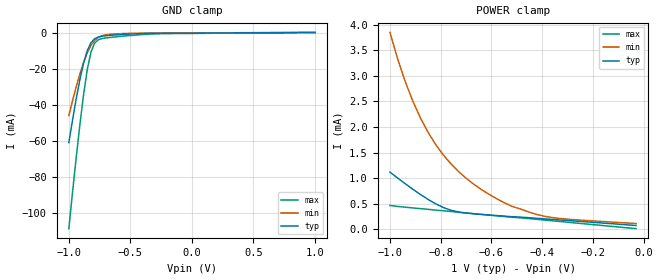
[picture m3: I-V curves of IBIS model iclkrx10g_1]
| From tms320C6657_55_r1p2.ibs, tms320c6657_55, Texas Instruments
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|   Model Cell iclkrx10g_1
|iclkrx10g_1  [08July11 revision 1.3]
[Model]   iclkrx10g_1
Model_type   Input
Polarity   Non-Inverting
Vinl =  1.15
Vinh =  1.25
C_comp   5.02654p   4.29394p   6.16252p
[Model Spec]
Vinl   1.15   1.15   1.15
Vinh   1.25   1.25   1.25
[Temperature Range]   25   125   -40
[Voltage Range]   1   0.9   1.1
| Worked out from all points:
|   GND clamp passes 1 mA (typ) near -0.56 V on its own axis
|   POWER clamp passes 1 mA (typ) near -0.97 V on its own axis
[GND_clamp]
|   voltage   I(typ)   I(min)   I(max)
-1V       -60.88mA   -45.91mA   -108.5mA
-940mV    -36.6mA    -29.97mA   -69.05mA
-910mV    -25.93mA   -22.84mA   -50.79mA
-880mV    -16.82mA   -16.48mA   -34.22mA
-850mV    -9.913mA   -11.15mA   -20.37mA
-820mV    -5.577mA   -7.06mA    -10.7mA
-790mV    -3.405mA   -4.281mA   -5.775mA
-760mV    -2.454mA   -2.625mA   -3.962mA
-700mV    -1.754mA   -1.25mA    -2.986mA
-640mV    -1.394mA   -811.8uA   -2.514mA
-300mV    -411.2uA   -270.4uA   -717.9uA
1V        64.27uA    104.3uA    -1.417uA
[POWER_clamp]
|   voltage   I(typ)   I(min)   I(max)
-1V       1.118mA    3.85mA     465.3uA
-970mV    1.004mA    3.34mA     447.5uA
-940mV    892.4uA    2.894mA    432.6uA
-910mV    784.7uA    2.509mA    418.3uA
-850mV    585.7uA    1.899mA    390.2uA
-820mV    499.2uA    1.66mA     376.2uA
-760mV    373uA      1.282mA    348.1uA
-670mV    303uA      883.6uA    306uA
-550mV    258.1uA    521.5uA    250uA
-420mV    214.9uA    288.2uA    194.1uA
-300mV    171.9uA    197.9uA    138.2uA
-30mV     75.02uA    113.1uA    12.54uA
